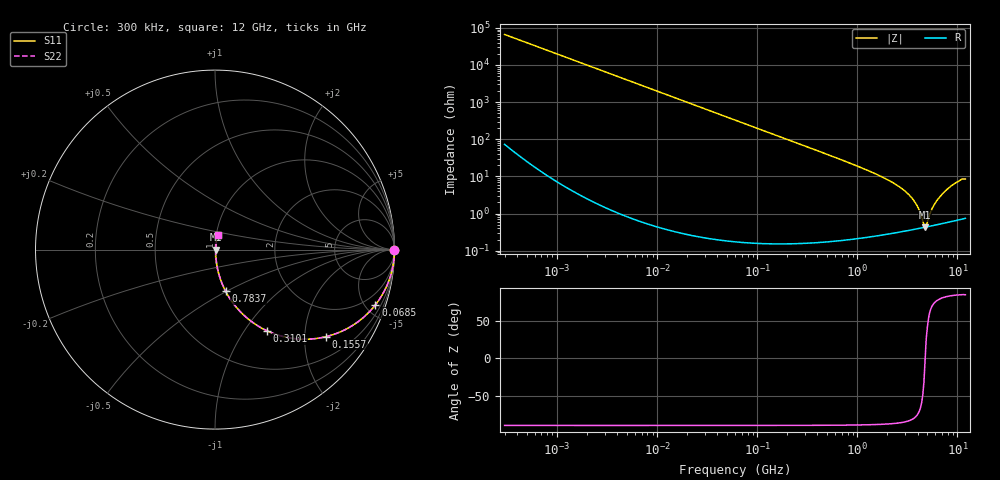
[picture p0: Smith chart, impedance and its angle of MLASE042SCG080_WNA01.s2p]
! MLASE042SCG080_WNA01  S-PARAMETER MODEL  ( General Type )
! Model Generated by TAIYO YUDEN Corporation (http://www.ty-top.com)
! Version 1.0
! TAIYO YUDEN Control No. 130801
! Copyright(c) 2013 TAIYO YUDEN CO.,LTD. All Rights Reserved.
! Product Description (link to TY-COMPAS)
! https://ds.yuden.co.jp/TYCOMPAS/or/detail?pn=MLASE042SCG080BWNA01&u=M
! Products Name : Multilayer Ceramic Capacitors
! Characteristics :
!  Capacitance : 8 pF , Rated Voltage : 16V , TCC : CG / C0G
!  Case Size : 0.4 x 0.2 / 0.016 x 0.008 [mm/inch] , Thickness : 0.2 / 0.008 [mm/inch]
!  (Conditions: Temperature = 25 degC , DC Bias Current/Voltage = 0A / 0V)
! External Node Assignments :
!  1  o---| |---o  2
! GND o---------o GND
! Frequency Range : 0.3MHz  -  12000MHz  [ 401 STEP ]
# MHz S RI R 50
! Freq[MHz].  S11 Real  S11 Imag  S21 Real  S21 Imag  S12 Real  S12 Imag  S22 Real  S22 Imag
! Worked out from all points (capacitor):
!   401 points, 300 kHz to 12 GHz, reference 50 ohm
!   read as one part in series: C = 8.01 pF near 316.3 kHz
!   lowest |Z| = 432 mohm at 4.748 GHz (marker M1)
!   series resonance near 4.764 GHz, so ESL is about 140 pH
!   S11 on the Smith chart (normalised r, x): 300 kHz: open; 68.5 MHz: 1.00, -5.80; 155.7 MHz: 1.00, -2.55; 310.1 MHz: 1.00, -1.28; 783.7 MHz: 1.00, -0.49; 12 GHz: 1.01, +0.17
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0.3  1 -0.00151  3.95e-06 0.00151  3.95e-06 0.00151  1 -0.00151
1.769972  0.9999 -0.00891  8.17e-05 0.00891  8.17e-05 0.00891  0.9999 -0.00891
10.44266  0.9972 -0.0524  0.00277 0.0524  0.00277 0.0524  0.9972 -0.0524
27.10171  0.9817 -0.1339  0.0183 0.1339  0.0183 0.1339  0.9817 -0.1339
60  0.9163 -0.2767  0.0837 0.2767  0.0837 0.2767  0.9163 -0.2767
68.49786  0.8936 -0.3081  0.1064 0.3081  0.1064 0.3081  0.8936 -0.3081
155.7172  0.6188 -0.4851  0.3812 0.4851  0.3812 0.4851  0.6188 -0.4851
310.0777  0.2898 -0.4524  0.7102 0.4524  0.7102 0.4524  0.2898 -0.4524
353.9943  0.2382 -0.4245  0.7618 0.4245  0.7618 0.4245  0.2382 -0.4245
783.7017  0.059 -0.2317  0.941 0.2317  0.941 0.2317  0.059 -0.2317
2088.533  0.00867 -0.076  0.9913 0.076  0.9913 0.076  0.00867 -0.076
2795.104  0.00541 -0.0463  0.9946 0.0463  0.9946 0.0463  0.00541 -0.0463
3454.93  0.00436 -0.0272  0.9956 0.0272  0.9956 0.0272  0.00436 -0.0272
3944.255  0.00413 -0.0159  0.9959 0.0159  0.9959 0.0159  0.00413 -0.0159
4502.883  0.00419 -0.00483  0.9958 0.00483  0.9958 0.00483  0.00419 -0.00483
4747.894  0.00429 -0.000315  0.9957 0.000315  0.9957 0.000315  0.00429 -0.000315
5006.236  0.00443 0.00392  0.9956 -0.00392  0.9956 -0.00392  0.00443 0.00392
5420.343  0.00472 0.0104  0.9953 -0.0104  0.9953 -0.0104  0.00472 0.0104
5868.704  0.00511 0.0168  0.9949 -0.0168  0.9949 -0.0168  0.00511 0.0168
6879.757  0.00623 0.0306  0.9938 -0.0306  0.9938 -0.0306  0.00623 0.0306
9207.246  0.0101 0.0613  0.9899 -0.0613  0.9899 -0.0613  0.0101 0.0613
12000  0.0144 0.0833  0.9856 -0.0833  0.9856 -0.0833  0.0144 0.0833
